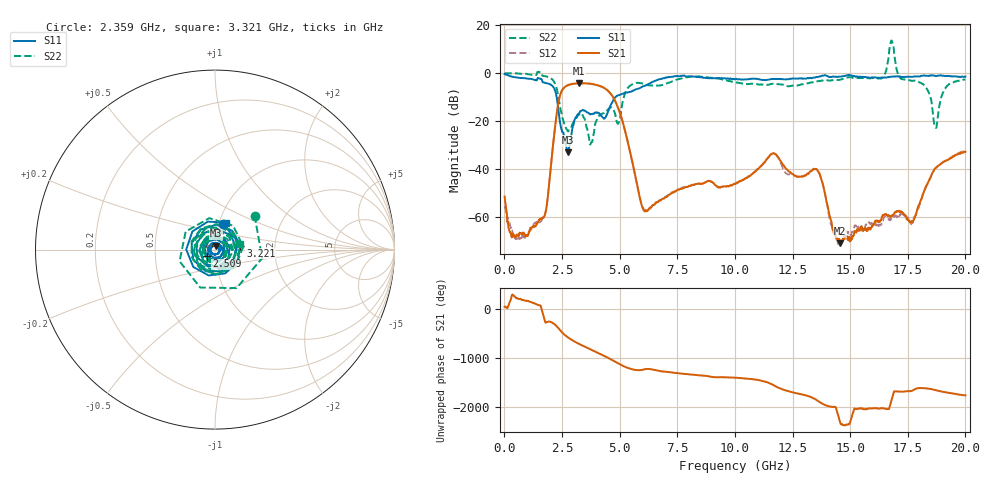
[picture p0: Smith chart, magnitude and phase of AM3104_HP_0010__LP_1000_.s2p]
!Created with skrf (http://scikit-rf.org).
# Hz S RI R 50.0
!freq ReS11 ImS11 ReS21 ImS21 ReS12 ImS12 ReS22 ImS22
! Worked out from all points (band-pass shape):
!   1601 points, 10 MHz to 20 GHz, reference 50 ohm
!   highest |S21| = -4.21 dB at 3.246 GHz (marker M1); lowest = -70.9 dB at 14.57 GHz (marker M2)
!   |S21| within 3 dB of the highest: 2.499 GHz to 4.481 GHz (1.982 GHz wide, 56.8 % of centre)
!   lowest |S11| = -33.0 dB at 2.759 GHz (marker M3), VSWR 1.05, Z = 50.7 + j2.14 ohm
!   |S11| at or under -10 dB: 2.269 GHz to 4.816 GHz (2.548 GHz wide, 71.9 % of centre)
!   |S22| runs from -29.8 to 13.7 dB; largest |S21 - S12| = 0.044
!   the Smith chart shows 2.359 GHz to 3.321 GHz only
!   S11 on the Smith chart (normalised r, x): 2.359 GHz: 1.05, +0.30; 2.509 GHz: 0.91, -0.07; 3.221 GHz: 1.33, +0.06; 3.321 GHz: 1.08, +0.33
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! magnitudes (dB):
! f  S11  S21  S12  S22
! 10 MHz  -0.4  -51.5  -55.5  -0.1
! 397.3 MHz  -1.6  -67.4  -67.7  -0.1
! 1.697 GHz  -3.9  -60.4  -60.4  -1.1
! 2.359 GHz  -16.5  -11.6  -11.6  -10.7
! 2.509 GHz  -24.5  -7.0  -7.1  -18.4
! 2.759 GHz  -33.0  -5.0  -5.0  -24.3
! 3.221 GHz  -16.9  -4.2  -4.3  -17.3
! 3.246 GHz  -16.8  -4.2  -4.3  -17.3
! 3.321 GHz  -15.8  -4.2  -4.3  -16.9
! 3.346 GHz  -15.7  -4.2  -4.3  -16.8
! 3.758 GHz  -17.1  -4.4  -4.5  -29.0
! 4.695 GHz  -11.8  -9.7  -9.8  -14.7
! 6.007 GHz  -5.5  -56.3  -56.3  -4.4
! 6.682 GHz  -2.7  -53.6  -53.4  -5.2
! 10.01 GHz  -2.5  -46.3  -46.5  -3.9
! 11.64 GHz  -2.4  -33.6  -33.5  -4.4
! 13.34 GHz  -2.1  -40.7  -40.6  -3.9
! 14.57 GHz  -1.4  -70.9  -70.4  -2.7
! 16.68 GHz  -1.6  -59.6  -61.0  7.3
! 17.7 GHz  -1.5  -62.1  -62.6  -3.2
! 18.7 GHz  -1.1  -39.7  -39.6  -22.6
! 20 GHz  -1.4  -32.8  -31.9  -2.6
